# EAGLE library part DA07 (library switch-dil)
DIL/CODE SWITCH
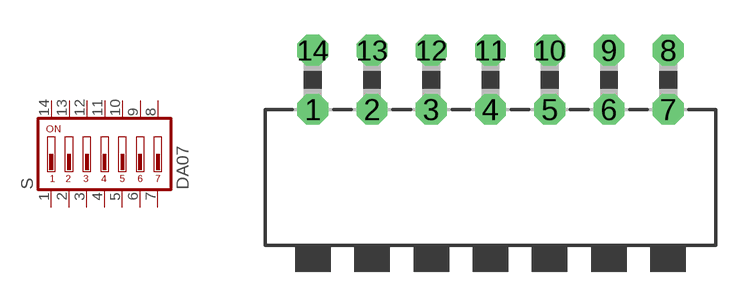
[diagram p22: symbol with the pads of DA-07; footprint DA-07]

Designator prefix S

## DA07 (MPN: MCDA07; OC_FARNELL: 1522002; OC_NEWARK: 74M2974)  [DA-07]
1  1  pas
2  2  pas
3  3  pas
4  4  pas
5  5  pas
6  6  pas
7  7  pas
8  8  pas
9  9  pas
10  10  pas
11  11  pas
12  12  pas
13  13  pas
14  14  pas

## Footprint DA-07 (pad centres in mm)
DIL/CODE SWITCH Mors distributor Buerklin, 17G590
drill 0.813 octagon: 1 -7.62,-1.27; 2 -5.08,-1.27; 3 -2.54,-1.27; 4 0,-1.27; 5 2.54,-1.27; 6 5.08,-1.27; 7 7.62,-1.27; 8 7.62,1.27; 9 5.08,1.27; 10 2.54,1.27; 11 0,1.27; 12 -2.54,1.27; 13 -5.08,1.27; 14 -7.62,1.27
